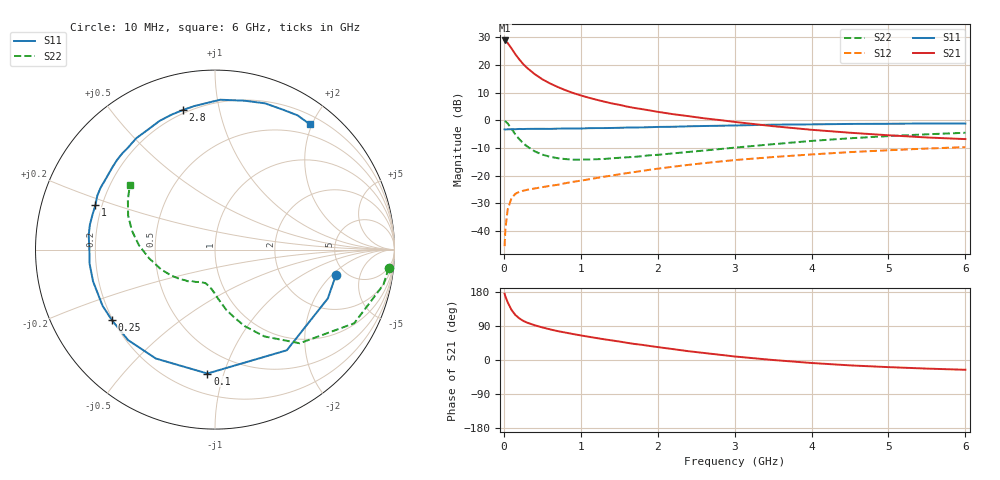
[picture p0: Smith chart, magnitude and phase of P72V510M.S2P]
! SIEMENS Small Signal Semiconductors
! BFP196
! Si NPN RF Bipolar Junction Transistor in SOT143
! VCE = 2.5 V  IC = 10 mA
! Common Emitter S-Parameters:  May  1996
# GHz  S  MA  R  50
!  f  S11  S21  S12  S22
! GHz  MAG  ANG  MAG  ANG  MAG  ANG  MAG  ANG
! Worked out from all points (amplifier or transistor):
!   36 points, 10 MHz to 6 GHz, reference 50 ohm
!   highest |S21| = 28.9 dB at 10 MHz (marker M1)
!   |S21| within 3 dB of that: start of sweep to 102.8 MHz
!   unconditionally stable (mu >= 1): 869.8 MHz to 3.308 GHz
!   at 250 MHz: K = 0.40, MSG = 22.9 dB, |S12| = -25.5 dB
!   at 1.4 GHz: K = 1.16, MAG = 10.7 dB, |S12| = -20.0 dB
!   at 6 GHz: K = 0.98, MSG = 1.4 dB, |S12| = -9.7 dB
!   S11 on the Smith chart (normalised r, x): 10 MHz: 4.12, -2.26; 100 MHz: 0.33, -0.88; 250 MHz: 0.20, -0.30; 1 GHz: 0.17, +0.18; 2.8 GHz: 0.18, +0.78; 6 GHz: 0.33, +1.97
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0.01  0.6882 -12.1  27.86 174.9  0.0053 86.2  0.9733 -6.1
0.02  0.685 -23.4  27.27 167.8  0.0108 80.0  0.9584 -11.8
0.05  0.6889 -54.5  25 152.2  0.0245 65.6  0.8775 -27.9
0.1  0.6918 -93.5  19.99 132.1  0.0393 50.0  0.7033 -47.9
0.15  0.6906 -118.5  15.67 118.7  0.0469 41.1  0.5563 -60.4
0.2  0.699 -133.8  12.69 110.0  0.051 36.1  0.4573 -68.8
0.25  0.6962 -145.5  10.48 103.5  0.0533 33.6  0.3871 -74.7
0.3  0.7004 -153.4  8.947 98.8  0.0553 32.9  0.3399 -79.5
0.4  0.7021 -165.4  6.872 91.8  0.0586 32.7  0.2758 -86.2
0.5  0.7031 -173.5  5.534 86.0  0.0619 33.4  0.2401 -91.0
0.6  0.7003 179.3  4.653 80.9  0.0653 35.1  0.2194 -95.3
0.7  0.7084 173.4  4.013 76.2  0.0683 36.5  0.2068 -99.2
0.8  0.7108 168.7  3.513 72.4  0.073 38.0  0.1993 -102.8
1  0.7113 159.4  2.823 64.9  0.0812 40.3  0.1947 -107.8
1.1  0.7215 155.3  2.578 61.4  0.0855 41.5  0.196 -110.6
1.6  0.7399 137.4  1.776 45.4  0.1111 44.0  0.2147 -124.2
2.2  0.7655 119.3  1.293 28.7  0.145 42.0  0.2525 -138.9
2.8  0.7982 102.9  1.014 14.0  0.1795 37.5  0.3017 -155.2
3.5  0.8355 88.0  0.784 0.0  0.2169 30.1  0.3704 -172.5
4.5  0.8613 71.1  0.597 -14.2  0.2664 19.3  0.474 167.3
5.5  0.8781 58.4  0.49 -22.7  0.3091 7.8  0.5596 150.2
6  0.8758 52.8  0.458 -25.8  0.3281 1.7  0.5963 142.6
